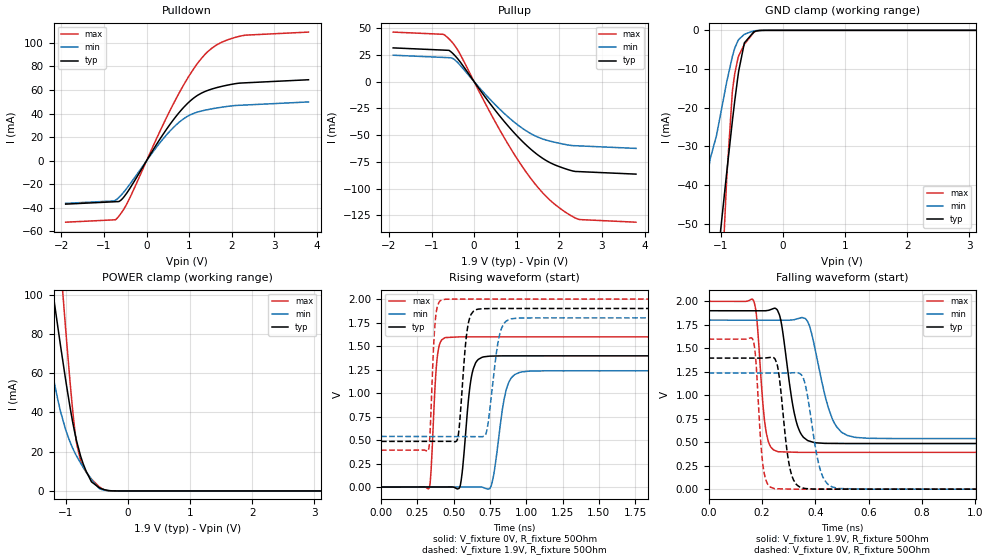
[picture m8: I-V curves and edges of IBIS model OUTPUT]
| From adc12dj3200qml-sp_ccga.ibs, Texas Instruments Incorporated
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||   Model OUTPUT
[Model]   OUTPUT
Model_type   3-state
Polarity   Non-Inverting
Vmeas = 0.95
Vref = 0
Cref = 5pF
Rref = 1e6
|   typ   min   max
C_comp   0.44pF   0.35pF   0.5pF
[Voltage Range]   1.9   1.8   2
[Temperature Range]   25   125   -40
[Pullup Reference]   1.9   1.8   2
[Pulldown Reference]   -0   0   0
[Power Clamp Reference]   1.9   1.8   2
[GND Clamp Reference]   0   0   0
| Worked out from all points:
|   slope of the pulldown table from 0 to 0.285 V, typ, clamps not added: 17 ohm
|   slope of the pullup table from 0 to 0.285 V, typ, clamps not added: 18.1 ohm
|   GND clamp passes 1 mA (typ) near -0.50 V on its own axis
|   POWER clamp passes 1 mA (typ) near -0.42 V on its own axis
|   falling waveform, V_fixture 1.9V, R_fixture 50Ohm: 20-80 % time 43.7ps typ, 63.4ps min, 25.8ps max; typ from 1.9 V to 0.486 V
|   rising waveform, V_fixture 0V, R_fixture 50Ohm: 20-80 % time 50ps typ, 67.9ps min, 31.5ps max; typ from 0 V to 1.4 V
|   rising waveform, V_fixture 1.9V, R_fixture 50Ohm: 20-80 % time 43.3ps typ, 60.5ps min, 27.3ps max; typ from 0.486 V to 1.9 V
|   falling waveform, V_fixture 0V, R_fixture 50Ohm: 20-80 % time 32.9ps typ, 43.5ps min, 21.7ps max; typ from 1.4 V to 0 V
[Pulldown]
|   Voltage   I(typ)   I(min)   I(max)
-1.9V     -36.85mA   -36.18mA   -52.16mA
-691.6mV  -34.73mA   -32.52mA   -48.81mA
-606.1mV  -33.58mA   -29.53mA   -44.89mA
-469.3mV  -27.68mA   -23.62mA   -37mA
248.9mV   14.71mA    12.26mA    19.94mA
647.9mV   35.58mA    28.79mA    49.51mA
893mV     46.08mA    36.12mA    65.68mA
1.127V    53.68mA    40.39mA    79.08mA
1.526V    60.69mA    43.92mA    95.21mA
1.845V    63.66mA    45.76mA    101.7mA
2.244V    65.89mA    47.08mA    106mA
3.8V      68.62mA    49.81mA    109mA
[GND Clamp]
|   Voltage   I(typ)   I(min)   I(max)
-1.9V     -277.6mA   -164.1mA   -535.1mA
-1.359V   -111.5mA   -56.84mA   -232mA
-1.279V   -92.67mA   -45.77mA   -188.2mA
-1.176V   -77.72mA   -33.41mA   -137.4mA
-1.062V   -60.41mA   -26.39mA   -91.83mA
-908.2mV  -36.88mA   -13.4mA    -38.52mA
-817mV    -23.55mA   -6.819mA   -15.95mA
-777.1mV  -18.11mA   -4.554mA   -11.14mA
-714.4mV  -10.53mA   -2.391mA   -6.587mA
-623.2mV  -3.245mA   -1.017mA   -3.611mA
-361mV    -39.38uA   -18.3uA    -21.12uA
3.8V      0A         0A         0A
[Pullup]
|   Voltage   I(typ)   I(min)   I(max)
-1.9V     31.54mA    24.69mA    46.3mA
-725.8mV  29.48mA    22.63mA    44.23mA
-560.5mV  28.43mA    22.35mA    38.79mA
-469.3mV  25.12mA    20.9mA     34.52mA
-349.6mV  19.6mA     16.31mA    27.15mA
408.5mV   -22.3mA    -18mA      -31.24mA
967.1mV   -48.98mA   -38.63mA   -69.4mA
1.48V     -67.99mA   -51.56mA   -97.98mA
1.925V    -78.26mA   -56.91mA   -115.6mA
2.244V    -82.7mA    -59.44mA   -124.5mA
2.472V    -84.08mA   -60.04mA   -128.9mA
3.8V      -86.41mA   -62.37mA   -131.3mA
[POWER Clamp]
|   Voltage   I(typ)   I(min)   I(max)
-1.9V     270.1mA    189.5mA    465.8mA
-1.393V   143.4mA    90.76mA    244.9mA
-1.199V   98.69mA    56.86mA    162.2mA
-1.085V   73.48mA    40.2mA     114.7mA
-1.011V   57.8mA     31.79mA    84.78mA
-896.8mV  35.95mA    22.15mA    42.75mA
-828.4mV  25.38mA    17.7mA     24.22mA
-720.1mV  13.6mA     12mA       11.91mA
-589mV    4.616mA    5.724mA    6.017mA
-452.2mV  1.487mA    1.085mA    1.814mA
-241.3mV  45.46uA    21.88uA    11.84uA
3.8V      0A         0A         0A
[Ramp]
R_load = 50
|   typ   min   max
dV/dt_r   0.83755/4.97388e-11   0.741902/6.73101e-11   0.958654/3.13718e-11
dV/dt_f   0.848685/4.35841e-11   0.756824/6.28978e-11   0.964669/2.57979e-11
[Falling Waveform]
V_fixture = 1.9V
V_fixture_min = 1.8V
V_fixture_max = 2V
R_fixture = 50Ohm
C_fixture = 0F
|   Time   V(typ)   V(min)   V(max)
0s        1.9V       1.8V       2V
168.7ps   1.9V       1.8V       2.007V
181ps     1.9V       1.8V       1.81V
215.1ps   1.9V       1.799V     622.7mV
259.3ps   1.899V     1.799V     399.7mV
327.9ps   729mV      1.81V      392.8mV
396.1ps   496.1mV    1.534V     392.3mV
467.2ps   486.8mV    728mV      392.3mV
552.5ps   485.6mV    550.7mV    392.3mV
3ns       485.5mV    538.6mV    392.2mV
[Rising Waveform]
V_fixture = 0V
V_fixture_min = 0V
V_fixture_max = 0V
R_fixture = 50Ohm
C_fixture = 0F
|   Time   V(typ)   V(min)   V(max)
0s        1.613uV    1.554uV    854.7nV
331.2ps   735.4uV    540.1uV    -9.643mV
385.4ps   855.7uV    628.4uV    1.355V
438.9ps   974.2uV    715.3uV    1.588V
543.3ps   4.128mV    885.1uV    1.598V
621ps     1.159V     1.011mV    1.598V
695.6ps   1.38V      -1.371mV   1.598V
759.3ps   1.393V     16.32mV    1.598V
951.3ps   1.396V     1.218V     1.598V
3ns       1.396V     1.237V     1.598V
[Rising Waveform]
V_fixture = 1.9V
V_fixture_min = 1.8V
V_fixture_max = 2V
R_fixture = 50Ohm
C_fixture = 0F
|   Time   V(typ)   V(min)   V(max)
0s        485.5mV    538.6mV    392.2mV
326ps     486mV      537.5mV    391.8mV
372.6ps   486mV      537.3mV    1.755V
417.8ps   486.1mV    537.2mV    1.991V
526.2ps   508.2mV    536.8mV    2V
594ps     1.677V     536.5mV    2V
658.8ps   1.889V     536.3mV    2V
726.3ps   1.898V     586.2mV    2V
889.9ps   1.9V       1.787V     2V
3ns       1.9V       1.8V       2V
[Falling Waveform]
|Gnd
V_fixture = 0V
V_fixture_min = 0V
V_fixture_max = 0V
R_fixture = 50Ohm
C_fixture = 0F
|   Time   V(typ)   V(min)   V(max)
0s        1.396V     1.237V     1.598V
165.6ps   1.396V     1.236V     1.596V
177.2ps   1.396V     1.236V     1.373V
205.6ps   1.395V     1.236V     219.4mV
246.7ps   1.393V     1.236V     5.825mV
306.8ps   199.7mV    1.238V     615.7uV
359.7ps   7.955mV    1.142V     32.3uV
418.2ps   848.5uV    210.5mV    31.6uV
485.4ps   75.35uV    8.08mV     30.8uV
3ns       1.616uV    1.566uV    855.7nV
